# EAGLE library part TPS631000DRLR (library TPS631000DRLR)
Switching Voltage Regulators 1.5-A output current, high power density buck-boost converter Source: Datasheet
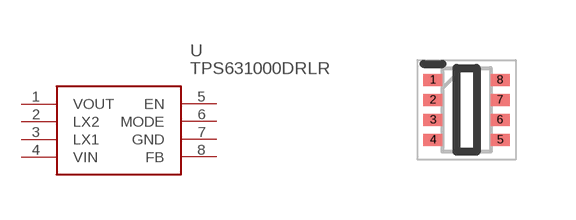
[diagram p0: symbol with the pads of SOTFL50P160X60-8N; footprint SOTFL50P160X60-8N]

Designator prefix U

## TPS631000DRLR (Description: Switching Voltage Regulators 1.5-A output current, high power density buck-boost converter; Height: 0.6mm; Manufacturer_Name: Texas Instruments; Manufacturer_Part_Number: TPS631000DRLR; Mouser_Part_Number: 595-TPS631000DRLR; Mouser_Price-Stock: https://www.mouser.co.uk/ProductDetail/Texas-Instruments/TPS631000DRLR?qs=rSMjJ%252B1ewcRYwoN2deTeNA%3D%3D)  [SOTFL50P160X60-8N]
1  VOUT
2  LX2
3  LX1
4  VIN
5  EN
6  MODE
7  GND
8  FB

## Footprint SOTFL50P160X60-8N (pad centres in mm)
DRL0008A
smd 0.475 x 0.3: 1 -0.838,0.75; 2 -0.838,0.25; 3 -0.838,-0.25; 4 -0.838,-0.75; 5 0.838,-0.75; 6 0.838,-0.25; 7 0.838,0.25; 8 0.838,0.75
